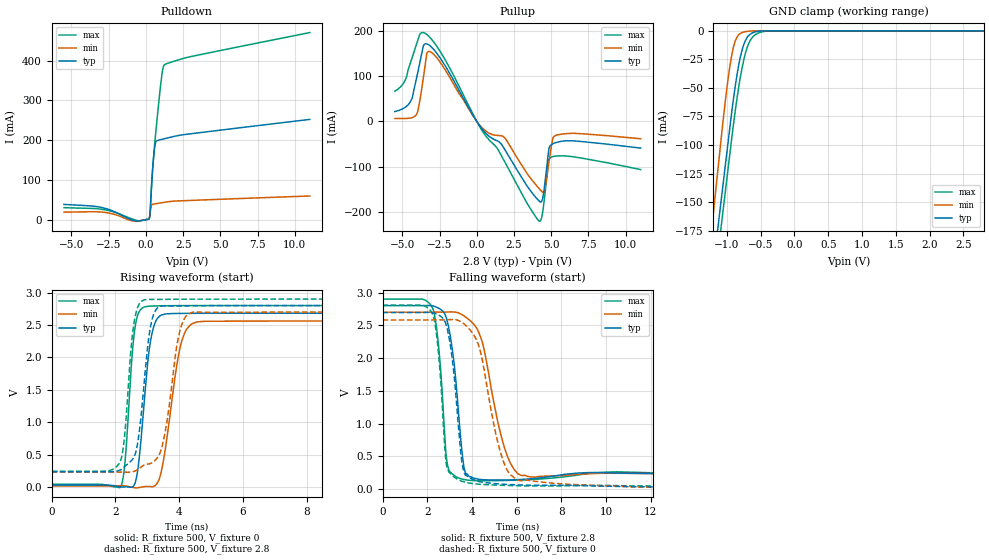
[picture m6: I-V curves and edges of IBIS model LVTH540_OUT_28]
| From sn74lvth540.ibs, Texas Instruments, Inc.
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[Model]   LVTH540_OUT_28
Model_type  3-state
Enable   Active-Low
Vref =   0
Rref =   500
Cref =   50p
Vmeas =   1.5
| variable   typ   min   max
C_comp   3.48pF   2.90pF   4.68pF
| C_pullup   3.98pF   0.17pF   5.57pF
| C_pulldown   4.62pF   0.13pF   12.18pF
| C_tri-state   3.48pF   2.90pF   4.68pF
[Temperature Range]   40   -40   100
| Ambient temperature   25   -40   85
[Voltage range]   2.8   2.7   2.9
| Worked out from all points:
|   slope of the pulldown table from 0 to 0.42 V, typ, clamps not added: 3.84 ohm
|   slope of the pullup table from 0 to 0.42 V, typ, clamps not added: 21.7 ohm
|   GND clamp passes 1 mA (typ) near -0.58 V on its own axis
|   rising waveform, R_fixture 500, V_fixture 0: 20-80 % time 300ps typ, 440ps min, 228ps max; typ from 0.032 V to 2.68 V
|   falling waveform, R_fixture 500, V_fixture 2.8: 20-80 % time 448ps typ, 885ps min, 341ps max; typ from 2.8 V to 0.238 V
|   rising waveform, R_fixture 500, V_fixture 2.8: 20-80 % time 321ps typ, 426ps min, 254ps max; typ from 0.238 V to 2.8 V
|   falling waveform, R_fixture 500, V_fixture 0: 20-80 % time 450ps typ, 902ps min, 344ps max; typ from 2.69 V to 0.032 V
[GND Clamp]
| LVTH540_OUT_28
|   Voltage   I(typ)   I(min)   I(max)
-5.5V     -2.834A    -3.019A    -2.854A
-1.22V    -215.7mA   -171mA     -239.3mA
-1.18V    -195.7mA   -148.2mA   -219mA
-1.075V   -143.6mA   -88.89mA   -166.6mA
-975mV    -94.01mA   -38.86mA   -117.1mA
-925mV    -69.63mA   -20.27mA   -92.47mA
-875mV    -47.88mA   -8.568mA   -69.46mA
-800mV    -22.55mA   -2.203mA   -40.18mA
-725mV    -8.33mA    -701.6uA   -19.48mA
-650mV    -2.727mA   -178.1uA   -7.97mA
-575mV    -842.6uA   -11.41uA   -3.176mA
2.8V      28.19pA    20.95pA    1.193nA
[Pulldown]
| LVTH540_OUT_28
|   Voltage   I(typ)   I(min)   I(max)
-5.5V     38.16mA    18.7mA     29.98mA
-2.92V    29.95mA    18.79mA    25.64mA
-690mV    -3.073mA   -4.361mA   -1.357mA
195mV     1.392mA    1.507mA    1.436mA
285mV     22.67mA    17.64mA    18.47mA
365mV     76.4mA     34.67mA    76.09mA
465mV     132.9mA    38.47mA    134.9mA
620mV     189.6mA    39.58mA    203.1mA
1.03V     201.6mA    42.25mA    352.1mA
1.135V    202.7mA    42.89mA    379.1mA
1.23V     203.6mA    43.45mA    389.4mA
11V       252.3mA    59.42mA    471mA
[Pullup]
| LVTH540_OUT_28
|   Voltage   I(typ)   I(min)   I(max)
-5.5V     21.77mA    6.604mA    66.92mA
-4.47V    42.68mA    7.356mA    128.3mA
-4.02V    99.38mA    17.02mA    173.5mA
-3.585V   167.5mA    96.63mA    196.9mA
-3.235V   170mA      155mA      189.3mA
140mV     -7.087mA   -6.066mA   -8.431mA
4.205V    -177mA     -149.5mA   -221.4mA
4.555V    -142mA     -152.3mA   -166.9mA
4.815V    -67.55mA   -96.73mA   -88.17mA
5V        -51.8mA    -56.89mA   -79.24mA
5.96V     -43.01mA   -27.21mA   -76.62mA
11V       -59.14mA   -38.42mA   -106.7mA
[Ramp]
| LVTH540_OUT_28
| variable   typ   min   max
dV/dt_r   1.61/3.11E-10   1.54/4.51E-10   1.69/2.34E-10
dV/dt_f   1.60/4.65E-10   1.51/9.13E-10   1.66/3.51E-10
R_load = 500
[Rising Waveform]
| LVTH540_OUT_28
R_fixture =   500
C_fixture =   0
L_fixture =   0
V_fixture =   0
V_fixture_min = 0
V_fixture_max = 0
|   Time   V(typ)   V(min)   V(max)
0s        32.2mV     19.9mV     45.21mV
2.17ns    368.2uV    20.5mV     12.32mV
2.3ns     4.953mV    18.74mV    397.3mV
2.62ns    69.9mV     -10.48mV   2.483V
2.75ns    471.3mV    -5.564mV   2.712V
3.045ns   2.067V     9.888mV    2.791V
3.435ns   2.654V     236.8mV    2.797V
4.08ns    2.68V      2.252V     2.8V
4.6ns     2.681V     2.551V     2.8V
50ns      2.684V     2.563V     2.801V
[Falling Waveform]
| LVTH540_OUT_28
R_fixture =   500
C_fixture =   0
L_fixture =   0
V_fixture =   2.8
V_fixture_min = 2.7
V_fixture_max = 2.9
|   Time   V(typ)   V(min)   V(max)
0s        2.8V       2.7V       2.9V
2.255ns   2.796V     2.701V     2.753V
2.525ns   2.758V     2.701V     2.115V
2.785ns   2.671V     2.702V     801.2mV
2.99ns    2.412V     2.704V     272.2mV
3.765ns   230.1mV    2.614V     140.1mV
4.465ns   145.4mV    2.236V     128.7mV
5.61ns    139.9mV    481.2mV    133.7mV
6.61ns    157.5mV    187.3mV    146.1mV
50ns      237.6mV    231.9mV    243.7mV
[Rising Waveform]
| LVTH540_OUT_28
R_fixture =   500
C_fixture =   0
L_fixture =   0
V_fixture =   2.8
V_fixture_min = 2.7
V_fixture_max = 2.9
|   Time   V(typ)   V(min)   V(max)
0s        238mV      232.1mV    244.1mV
2.135ns   259.6mV    231.4mV    374.8mV
2.28ns    311.6mV    231.2mV    759.2mV
2.58ns    465.7mV    242.8mV    2.526V
2.925ns   1.753V     344.2mV    2.892V
3.285ns   2.747V     435.1mV    2.897V
3.56ns    2.796V     852.7mV    2.897V
4.02ns    2.796V     2.411V     2.899V
4.44ns    2.798V     2.699V     2.899V
50ns      2.8V       2.7V       2.9V
[Falling Waveform]
| LVTH540_OUT_28
R_fixture =   500
C_fixture =   0
L_fixture =   0
V_fixture =   0
V_fixture_min = 0
V_fixture_max = 0
|   Time   V(typ)   V(min)   V(max)
0s        2.695V     2.582V     2.808V
2.255ns   2.691V     2.583V     2.659V
2.515ns   2.656V     2.583V     2.028V
2.765ns   2.576V     2.584V     736.2mV
3.125ns   1.965V     2.588V     207.1mV
3.56ns    393.1mV    2.542V     120.1mV
3.895ns   172.9mV    2.438V     91.41mV
5.36ns    76.49mV    466.6mV    58.83mV
6.14ns    64.4mV     129.9mV    51.9mV
50ns      32.23mV    19.91mV    45.26mV
